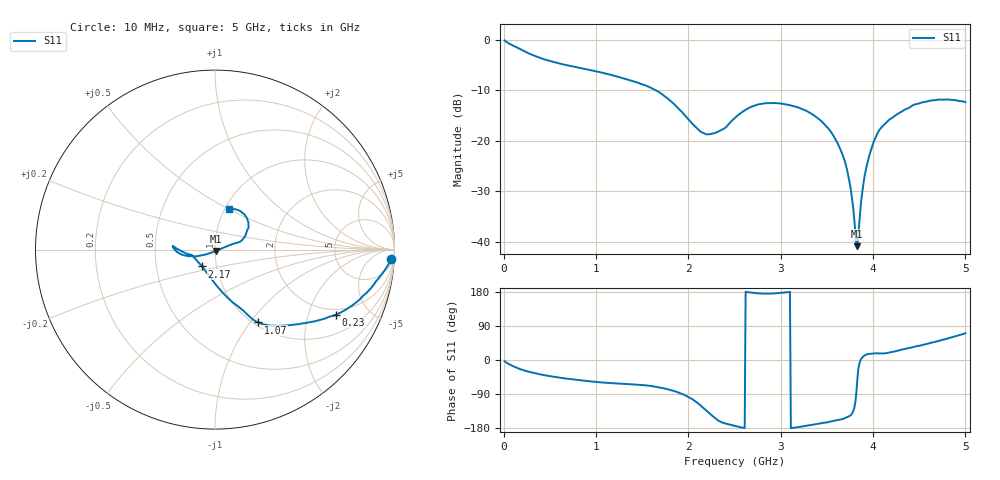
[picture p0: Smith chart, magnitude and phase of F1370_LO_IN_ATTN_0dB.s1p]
! S-parameters for LO input IDT F1370 DPD Demodulator
! Date Measured:  2015-11-25  RGG
!  Port 1 = Pin 12 = LO_IN
! State: 0 dB attenuation (Gain = Gmax - 0 dB)
! LO Frequency:  10 MHz to 5000 MHz
! RF_INX, RF_INY, IF_I+, IF_I-, IF_Q+, and IF_Q- terminated
! Vcc = +5.00 Volts  Icc = approx 275 mA.
! NOTES:  The device was measured on a custom printed circuit evaluation board with individual 50 ohm
!  microstrip lines to the RF and LO pins. The 50 ohm microstrip lines were de-embedded using reference
!  plane extensions
! Frequency Re{S11} Im{S11}
# HZ  S  RI R 50.00
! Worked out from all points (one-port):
!   500 points, 10 MHz to 5 GHz, reference 50 ohm
!   lowest |S11| = -40.8 dB at 3.83 GHz (marker M1), VSWR 1.02, Z = 50.6 - j0.718 ohm
!   |S11| at or under -10 dB: 1.647 GHz to end of sweep
!   S11 on the Smith chart (normalised r, x): 10 MHz: 11, -34; 230 MHz: 1.74, -3.05; 1.07 GHz: 1.05, -1.09; 2.17 GHz: 0.85, -0.16; 5 GHz: 1.05, +0.51
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1e7  0.982 -0.0521
1.1e8  0.8251 -0.2569
2.3e8  0.6737 -0.3624
4e8  0.5175 -0.4062
6.4e8  0.3835 -0.4239
1.07e9  0.2403 -0.4057
1.26e9  0.1961 -0.3765
1.65e9  0.1031 -0.2978
1.89e9  0.0164 -0.2095
2.17e9  -0.0734 -0.0937
2.37e9  -0.1257 -0.033
2.51e9  -0.1702 -0.0172
2.77e9  -0.2298 0.0168
3.13e9  -0.2213 -0.00296
3.35e9  -0.1792 -0.0301
3.55e9  -0.1145 -0.0375
3.68e9  -0.0622 -0.029
3.76e9  -0.0268 -0.0186
3.81e9  -0.00368 -0.0109
3.83e9  0.00571 -0.00709
3.84e9  0.0102 -0.00472
3.88e9  0.0294 0.00285
3.91e9  0.0447 0.00966
4.01e9  0.095 0.0298
4.14e9  0.1434 0.0464
4.38e9  0.1796 0.1098
4.7e9  0.1657 0.1944
5e9  0.0797 0.2278
